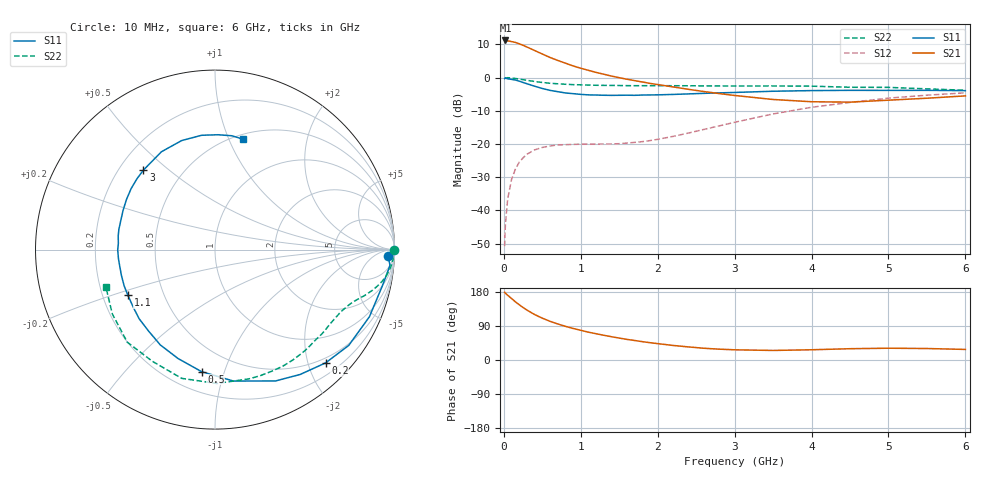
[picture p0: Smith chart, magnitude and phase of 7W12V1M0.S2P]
! Infineon Technologies  Discrete & RF Semiconductors
! BFS17W
! Si NPN RF Bipolar Junction Transistor in SOT323
! VCE = 12 V  IC = 1 mA
! Common Emitter S-Parameters:  August  1999
# GHz  S  MA  R  50
!  f  S11  S21  S12  S22
! GHz  MAG  ANG  MAG  ANG  MAG  ANG  MAG  ANG
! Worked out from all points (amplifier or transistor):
!   36 points, 10 MHz to 6 GHz, reference 50 ohm
!   highest |S21| = 11.2 dB at 20 MHz (marker M1)
!   |S21| within 3 dB of that: start of sweep to 397.8 MHz
!   unconditionally stable (mu >= 1): 1.088 GHz to 2.993 GHz; 4.158 GHz to end of sweep
!   at 250 MHz: K = 0.25, MSG = 16.9 dB, |S12| = -24.2 dB
!   at 1.4 GHz: K = 1.21, MAG = 7.4 dB, |S12| = -20.0 dB
!   at 6 GHz: K = 1.08, MAG = -2.2 dB, |S12| = -4.6 dB
!   S11 on the Smith chart (normalised r, x): 10 MHz: 26, -27; 200 MHz: 0.41, -2.31; 500 MHz: 0.33, -0.84; 1.1 GHz: 0.31, -0.22; 3 GHz: 0.30, +0.41; 6 GHz: 0.55, +1.13
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0.01  0.9639 -2.2  3.588 178.8  0.0029 84.3  0.9999 -0.1
0.02  0.9792 -5.1  3.61 176.4  0.0061 93.4  0.9831 -1.1
0.05  0.9548 -12.0  3.569 170.8  0.0149 81.7  0.9941 -3.0
0.1  0.9382 -23.5  3.472 162.4  0.0292 75.7  0.9835 -5.8
0.15  0.9166 -35.6  3.375 153.6  0.0418 69.8  0.9668 -8.5
0.2  0.8821 -45.7  3.217 145.8  0.0532 65.4  0.9483 -10.7
0.25  0.842 -55.7  3.052 138.5  0.0618 59.7  0.927 -12.7
0.3  0.806 -65.2  2.877 131.8  0.0701 55.3  0.9072 -14.4
0.4  0.7397 -82.0  2.549 120.0  0.0816 48.1  0.8716 -17.1
0.5  0.684 -96.3  2.257 110.4  0.0886 43.5  0.8417 -19.2
0.6  0.6409 -108.7  2.004 102.1  0.0933 39.9  0.8199 -21.0
0.7  0.6124 -119.8  1.809 95.1  0.0967 38.3  0.8045 -22.8
0.8  0.5857 -129.2  1.644 88.9  0.0976 36.9  0.7917 -24.7
1.1  0.5479 -152.4  1.282 73.4  0.1 37.5  0.7695 -30.2
1.6  0.542 -179.8  0.942 54.4  0.1031 47.4  0.7543 -40.7
2.2  0.5565 157.1  0.722 38.4  0.13 64.5  0.7525 -54.9
3  0.596 132.0  0.537 26.9  0.2119 73.6  0.7446 -75.2
3.5  0.6215 118.7  0.467 25.2  0.2832 71.8  0.746 -89.2
4  0.6353 107.0  0.432 27.0  0.3568 66.5  0.741 -104.5
4.5  0.6413 96.7  0.426 29.8  0.4217 59.7  0.7134 -119.4
5.5  0.6412 81.5  0.488 30.3  0.5419 45.3  0.675 -148.0
6  0.6346 75.8  0.529 27.9  0.588 38.4  0.6428 -160.9
